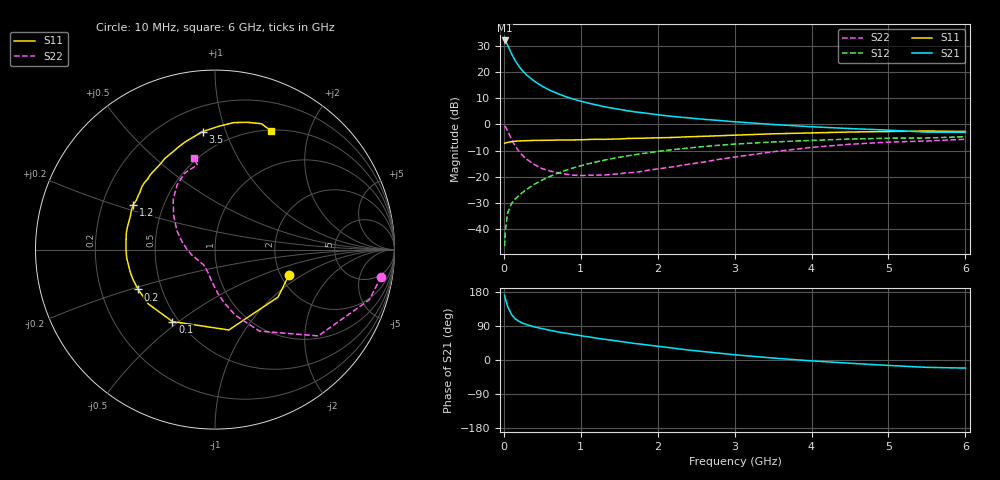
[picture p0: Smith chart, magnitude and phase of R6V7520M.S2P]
! SIEMENS Small Signal Semiconductors
! BFR193
! Si NPN RF Bipolar Junction Transistor in SOT23
! VCE = 0.75 V  IC = 20 mA
! Common Emitter S-Parameters:  May  1996
# GHz  S  MA  R  50
!  f  S11  S21  S12  S22
! GHz  MAG  ANG  MAG  ANG  MAG  ANG  MAG  ANG
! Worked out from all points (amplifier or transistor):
!   36 points, 10 MHz to 6 GHz, reference 50 ohm
!   highest |S21| = 32.1 dB at 10 MHz (marker M1)
!   |S21| within 3 dB of that: start of sweep to 68.1 MHz
!   unconditionally stable (mu >= 1): 478.4 MHz to 2.303 GHz
!   at 250 MHz: K = 0.85, MSG = 23.1 dB, |S12| = -25.8 dB
!   at 1.4 GHz: K = 1.04, MAG = 8.5 dB, |S12| = -13.1 dB
!   at 6 GHz: K = 0.99, MSG = 0.8 dB, |S12| = -4.7 dB
!   S11 on the Smith chart (normalised r, x): 10 MHz: 2.20, -0.78; 100 MHz: 0.46, -0.47; 200 MHz: 0.37, -0.21; 1.2 GHz: 0.33, +0.23; 3.5 GHz: 0.36, +0.83; 6 GHz: 0.51, +1.46
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0.01  0.4354 -19.3  40.28 170.9  0.0047 81.0  0.9378 -9.2
0.02  0.4397 -37.0  39.03 162.0  0.0096 77.4  0.9043 -18.0
0.05  0.4545 -80.2  32.68 140.7  0.0205 64.8  0.7498 -39.9
0.1  0.4657 -120.6  22.42 119.9  0.0306 58.4  0.5173 -61.4
0.15  0.4789 -140.7  16.34 108.4  0.0378 57.6  0.3825 -72.8
0.2  0.4824 -152.6  12.73 101.6  0.0439 59.4  0.3007 -80.2
0.25  0.4867 -160.4  10.33 96.7  0.0511 60.9  0.2486 -85.8
0.3  0.4887 -165.7  8.713 93.1  0.0577 62.8  0.2145 -89.8
0.4  0.4944 -174.9  6.64 87.4  0.0722 64.7  0.17 -97.3
0.5  0.4962 179.5  5.343 82.6  0.0866 65.7  0.1426 -103.8
0.6  0.498 174.3  4.487 78.3  0.1016 65.9  0.1283 -109.1
0.7  0.5028 169.5  3.877 74.2  0.1166 65.7  0.1193 -114.2
0.9  0.5048 161.5  3.058 67.4  0.1472 64.3  0.1072 -125.3
1.1  0.5146 154.6  2.549 61.0  0.177 62.2  0.1071 -134.6
1.2  0.5196 151.1  2.36 57.9  0.1917 61.1  0.1072 -139.6
1.7  0.5421 136.2  1.74 43.6  0.2631 54.0  0.1208 -161.4
2.2  0.5631 123.6  1.417 31.4  0.3296 46.2  0.1549 -180.0
3  0.6228 105.4  1.123 13.8  0.4202 33.1  0.2376 153.4
3.5  0.6613 96.0  0.998 5.2  0.4612 25.0  0.3001 140.2
4.5  0.7154 81.6  0.833 -8.6  0.5244 11.0  0.4178 120.3
5.5  0.7476 69.8  0.711 -19.4  0.5499 -2.3  0.4823 101.8
6  0.7316 64.6  0.705 -21.3  0.582 -6.3  0.5206 102.8
